FUNCTION_BLOCK FB_Mathematics
VAR_INPUT
END_VAR
VAR_OUTPUT
END_VAR
VAR
	{attribute 'OPC.UA.DA':='1'}
	nNumberOfCallsMMul : INT;
END_VAR

{attribute 'TcRpcEnable':='1'}
METHOD M_Mul : DINT
VAR_INPUT
	a : INT;
	b : INT;
END_VAR
M_Mul := a * b;
nNumberOfCallsMMul := nNumberOfCallsMMul + 1;
END_METHOD

END_FUNCTION_BLOCK
